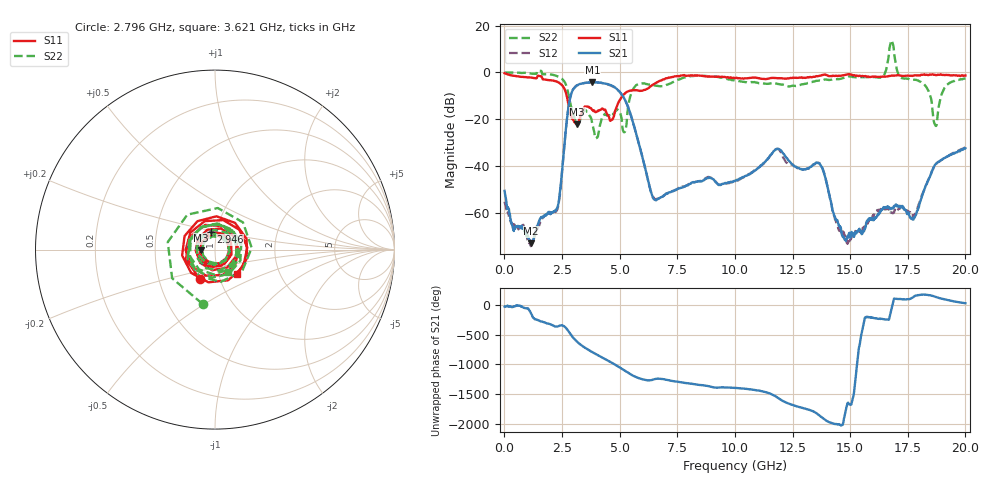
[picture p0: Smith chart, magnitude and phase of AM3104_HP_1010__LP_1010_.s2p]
!Created with skrf (http://scikit-rf.org).
# Hz S RI R 50.0
!freq ReS11 ImS11 ReS21 ImS21 ReS12 ImS12 ReS22 ImS22
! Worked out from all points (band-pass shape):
!   1601 points, 10 MHz to 20 GHz, reference 50 ohm
!   highest |S21| = -4.21 dB at 3.821 GHz (marker M1); lowest = -73.2 dB at 1.159 GHz (marker M2)
!   |S21| within 3 dB of the highest: 2.989 GHz to 4.888 GHz (1.899 GHz wide, 48.2 % of centre)
!   lowest |S11| = -22.2 dB at 3.158 GHz (marker M3), VSWR 1.17, Z = 42.8 - j0.356 ohm
!   |S11| at or under -10 dB: 2.703 GHz to 5.134 GHz (2.431 GHz wide, 62 % of centre)
!   |S22| runs from -28.3 to 13.6 dB; largest |S21 - S12| = 0.05
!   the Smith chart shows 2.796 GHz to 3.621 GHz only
!   S11 on the Smith chart (normalised r, x): 2.796 GHz: 0.80, -0.27; 2.946 GHz: 0.94, +0.19; 3.621 GHz: 1.22, -0.35
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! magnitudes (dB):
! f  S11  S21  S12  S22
! 10 MHz  -0.4  -50.7  -55.4  0.0
! 1.159 GHz  -2.2  -73.2  -74.3  -0.6
! 2.309 GHz  -4.1  -57.7  -58.5  -1.7
! 2.796 GHz  -14.7  -13.9  -13.9  -10.2
! 2.946 GHz  -19.9  -8.0  -8.1  -16.6
! 3.158 GHz  -22.2  -5.5  -5.6  -22.7
! 3.346 GHz  -17.6  -4.8  -4.9  -18.4
! 3.621 GHz  -14.7  -4.4  -4.5  -17.0
! 3.821 GHz  -16.1  -4.2  -4.2  -22.6
! 5.182 GHz  -9.4  -10.9  -10.9  -25.6
! 5.657 GHz  -7.7  -24.0  -24.1  -6.2
! 6.682 GHz  -4.0  -54.1  -54.1  -5.9
! 10.01 GHz  -2.5  -46.6  -46.7  -3.6
! 11.82 GHz  -2.5  -32.8  -32.8  -4.9
! 13.34 GHz  -2.1  -40.1  -40.1  -4.2
! 13.78 GHz  -1.2  -40.7  -40.5  -3.3
! 14.89 GHz  -0.9  -70.0  -73.3  -1.9
! 16.68 GHz  -1.6  -58.0  -58.7  7.2
! 17.76 GHz  -1.3  -62.2  -61.4  -3.2
! 18.69 GHz  -1.1  -39.5  -39.6  -22.5
! 19.13 GHz  -1.2  -36.6  -36.5  -6.4
! 20 GHz  -1.4  -32.5  -32.2  -2.6
